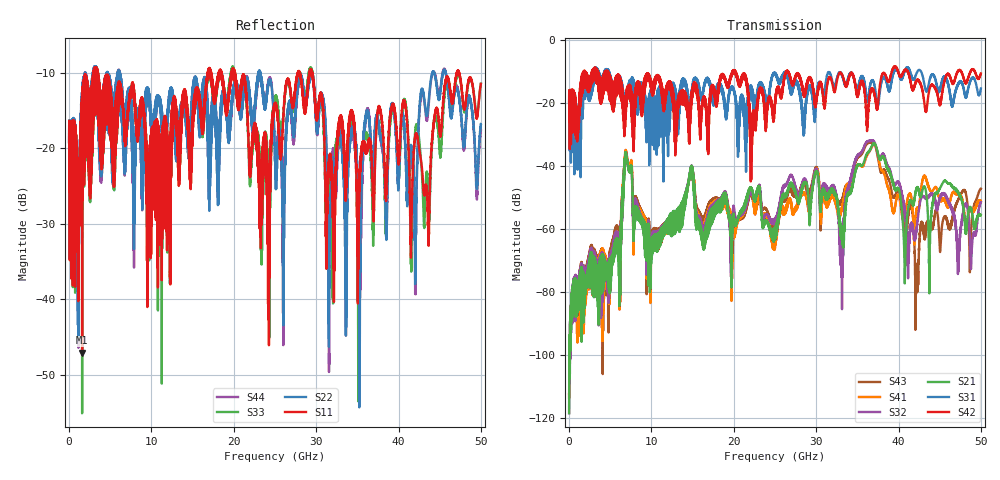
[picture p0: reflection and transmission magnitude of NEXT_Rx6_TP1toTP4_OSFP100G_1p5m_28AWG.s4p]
! Touchstone data
! Created: 27-Feb-2019 by IdEM 12 (12.1.0)
! COMMENTS
!  Created Wed Feb 27 09:43:39 2019
!  64 Port Network Data from SP1.SP block
!  freq  magS1_1  angS1_1  magS1_2  angS1_2  magS1_3  angS1_3  magS1_4  angS1_4
!  magS1_5  angS1_5  magS1_6  angS1_6  magS1_7  angS1_7  magS1_8  angS1_8
!  magS1_9  angS1_9  magS1_10  angS1_10  magS1_11  angS1_11  magS1_12  angS1_12
!  magS1_13  angS1_13  magS1_14  angS1_14  magS1_15  angS1_15  magS1_16  angS1_16
!  magS1_17  angS1_17  magS1_18  angS1_18  magS1_19  angS1_19  magS1_20  angS1_20
!  magS1_21  angS1_21  magS1_22  angS1_22  magS1_23  angS1_23  magS1_24  angS1_24
!  magS1_25  angS1_25  magS1_26  angS1_26  magS1_27  angS1_27  magS1_28  angS1_28
!  magS1_29  angS1_29  magS1_30  angS1_30  magS1_31  angS1_31  magS1_32  angS1_32
!  magS1_33  angS1_33  magS1_34  angS1_34  magS1_35  angS1_35  magS1_36  angS1_36
!  magS1_37  angS1_37  magS1_38  angS1_38  magS1_39  angS1_39  magS1_40  angS1_40
!  magS1_41  angS1_41  magS1_42  angS1_42  magS1_43  angS1_43  magS1_44  angS1_44
!  magS1_45  angS1_45  magS1_46  angS1_46  magS1_47  angS1_47  magS1_48  angS1_48
!  magS1_49  angS1_49  magS1_50  angS1_50  magS1_51  angS1_51  magS1_52  angS1_52
!  magS1_53  angS1_53  magS1_54  angS1_54  magS1_55  angS1_55  magS1_56  angS1_56
!  magS1_57  angS1_57  magS1_58  angS1_58  magS1_59  angS1_59  magS1_60  angS1_60
!  magS1_61  angS1_61  magS1_62  angS1_62  magS1_63  angS1_63  magS1_64  angS1_64
!  magS2_1  angS2_1  magS2_2  angS2_2  magS2_3  angS2_3  magS2_4  angS2_4
!  magS2_5  angS2_5  magS2_6  angS2_6  magS2_7  angS2_7  magS2_8  angS2_8
!  magS2_9  angS2_9  magS2_10  angS2_10  magS2_11  angS2_11  magS2_12  angS2_12
!  magS2_13  angS2_13  magS2_14  angS2_14  magS2_15  angS2_15  magS2_16  angS2_16
!  magS2_17  angS2_17  magS2_18  angS2_18  magS2_19  angS2_19  magS2_20  angS2_20
!  magS2_21  angS2_21  magS2_22  angS2_22  magS2_23  angS2_23  magS2_24  angS2_24
!  magS2_25  angS2_25  magS2_26  angS2_26  magS2_27  angS2_27  magS2_28  angS2_28
!  magS2_29  angS2_29  magS2_30  angS2_30  magS2_31  angS2_31  magS2_32  angS2_32
!  magS2_33  angS2_33  magS2_34  angS2_34  magS2_35  angS2_35  magS2_36  angS2_36
!  magS2_37  angS2_37  magS2_38  angS2_38  magS2_39  angS2_39  magS2_40  angS2_40
!  magS2_41  angS2_41  magS2_42  angS2_42  magS2_43  angS2_43  magS2_44  angS2_44
!  magS2_45  angS2_45  magS2_46  angS2_46  magS2_47  angS2_47  magS2_48  angS2_48
!  magS2_49  angS2_49  magS2_50  angS2_50  magS2_51  angS2_51  magS2_52  angS2_52
!  magS2_53  angS2_53  magS2_54  angS2_54  magS2_55  angS2_55  magS2_56  angS2_56
!  magS2_57  angS2_57  magS2_58  angS2_58  magS2_59  angS2_59  magS2_60  angS2_60
!  magS2_61  angS2_61  magS2_62  angS2_62  magS2_63  angS2_63  magS2_64  angS2_64
!  magS3_1  angS3_1  magS3_2  angS3_2  magS3_3  angS3_3  magS3_4  angS3_4
!  magS3_5  angS3_5  magS3_6  angS3_6  magS3_7  angS3_7  magS3_8  angS3_8
!  magS3_9  angS3_9  magS3_10  angS3_10  magS3_11  angS3_11  magS3_12  angS3_12
!  magS3_13  angS3_13  magS3_14  angS3_14  magS3_15  angS3_15  magS3_16  angS3_16
!  magS3_17  angS3_17  magS3_18  angS3_18  magS3_19  angS3_19  magS3_20  angS3_20
!  magS3_21  angS3_21  magS3_22  angS3_22  magS3_23  angS3_23  magS3_24  angS3_24
!  magS3_25  angS3_25  magS3_26  angS3_26  magS3_27  angS3_27  magS3_28  angS3_28
!  magS3_29  angS3_29  magS3_30  angS3_30  magS3_31  angS3_31  magS3_32  angS3_32
!  magS3_33  angS3_33  magS3_34  angS3_34  magS3_35  angS3_35  magS3_36  angS3_36
!  magS3_37  angS3_37  magS3_38  angS3_38  magS3_39  angS3_39  magS3_40  angS3_40
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# Hz S MA R 50
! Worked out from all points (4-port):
!   5000 points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, 10 MHz to 50 GHz, reference 50 ohm
!   strongest paths, dB at 10 MHz, 12.51 GHz, 25.01 GHz, 37.51 GHz, 50 GHz:
!     S42: -19.6, -16.4, -19.1, -20.0, -10.6
!     S31: -19.6, -16.2, -10.8, -21.0, -15.4
!     S21: -118.4, -59.4, -62.4, -36.0, -55.5
!     S32: -118.5, -59.4, -57.9, -36.4, -51.5
!     S41: -112.4, -58.9, -62.4, -36.6, -51.1
!     S43: -113.5, -58.8, -59.0, -37.5, -47.1
!   lowest |S11| = -47.1 dB at 1.59 GHz (marker M1), VSWR 1.01, Z = 49.7 + j0.298 ohm
!   |S11| at or under -10 dB: 3.482 GHz to 16.85 GHz (13.37 GHz wide, 132 % of centre); 20.15 GHz to 27.79 GHz (7.635 GHz wide, 31.9 % of centre); 29.53 GHz to 47.08 GHz (17.55 GHz wide, 45.8 % of centre)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
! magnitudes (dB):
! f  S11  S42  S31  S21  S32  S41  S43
! 10 MHz  -19.2  -19.6  -19.6  -118.4  -118.5  -112.4  -113.5
! 1.59 GHz  -47.1  -16.9  -24.2  -75.2  -73.0  -76.0  -72.9
! 6.95 GHz  -18.5  -18.7  -20.2  -36.3  -36.8  -35.8  -36.3
! 33.08 GHz  -16.7  -10.6  -10.6  -60.7  -65.9  -53.7  -51.6
! 36.85 GHz  -25.1  -15.3  -12.7  -33.2  -31.9  -33.6  -32.4
! 42.21 GHz  -18.2  -13.0  -10.4  -47.1  -59.6  -53.7  -71.2
! 50 GHz  -11.5  -10.6  -15.4  -55.5  -51.5  -51.1  -47.1
